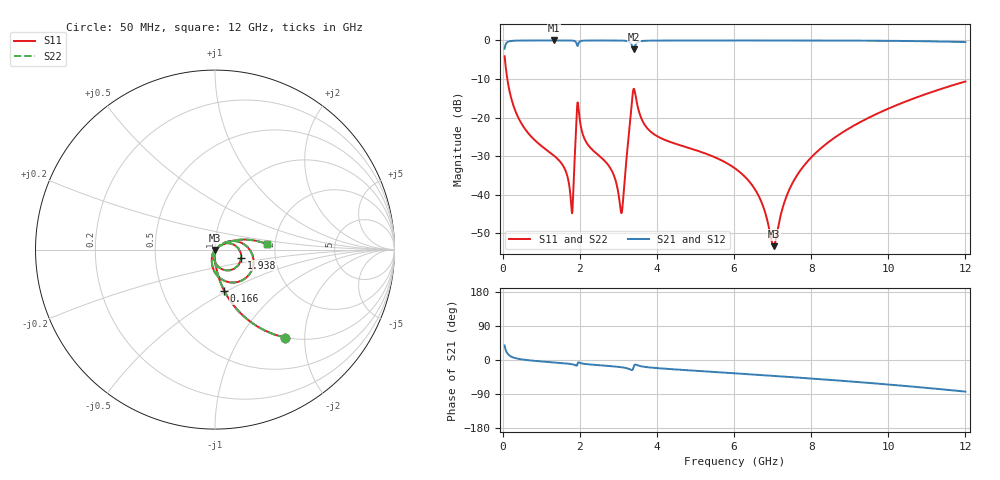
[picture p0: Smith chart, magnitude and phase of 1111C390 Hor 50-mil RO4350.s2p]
# GHz S MA R 50
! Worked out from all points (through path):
!   11951 points, 50 MHz to 12 GHz, reference 50 ohm
!   highest |S21| = -0.01 dB at 1.339 GHz (marker M1); lowest = -2.3 dB at 3.394 GHz (marker M2)
!   group delay of S21, straight-line fit = 19.6 ps
!   lowest |S11| = -53.3 dB at 7.025 GHz (marker M3), VSWR 1.00, Z = 50.2 - j0.147 ohm
!   |S11| at or under -10 dB: 120.3 MHz to end of sweep
!   |S22| runs from -53.3 to -4.1 dB; largest |S21 - S12| = 0
!   S11 on the Smith chart (normalised r, x): 50 MHz: 0.99, -1.59; 166 MHz: 0.99, -0.48; 1.938 GHz: 1.34, -0.12; 12 GHz: 1.82, +0.12
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0.05  0.6251 -51.6  0.7804 38.4  0.7804 38.4  0.6251 -51.6
0.166  0.2351 -77.4  0.9716 12.6  0.9716 12.6  0.2351 -77.4
0.549  0.07494 -88.8  0.9966 0.8  0.9966 0.8  0.07494 -88.8
1.339  0.03189 -95.0  0.9985 -6.6  0.9985 -6.6  0.03189 -95.0
1.624  0.02094 -94.7  0.9981 -9.0  0.9981 -9.0  0.02094 -94.7
1.786  0.006508 -55.1  0.9952 -10.9  0.9952 -10.9  0.006508 -55.1
1.832  0.01139 27.1  0.991 -11.9  0.991 -11.9  0.01139 27.1
1.938  0.1535 -17.1  0.847 -11.2  0.847 -11.2  0.1535 -17.1
2.042  0.07096 -89.1  0.9855 -8.8  0.9855 -8.8  0.07096 -89.1
2.827  0.02066 -99.6  0.9972 -16.4  0.9972 -16.4  0.02066 -99.6
3.074  0.005872 -40.8  0.9944 -19.0  0.9944 -19.0  0.005872 -40.8
3.125  0.008987 15.6  0.9925 -19.7  0.9925 -19.7  0.008987 15.6
3.394  0.2342 -26.9  0.7672 -19.3  0.7672 -19.3  0.2342 -26.9
3.662  0.08397 -101.3  0.9866 -17.9  0.9866 -17.9  0.08397 -101.3
4.034  0.05648 -108.4  0.9949 -21.7  0.9949 -21.7  0.05648 -108.4
6.025  0.02203 -120.0  0.9974 -35.2  0.9974 -35.2  0.02203 -120.0
6.629  0.009901 -117.1  0.9975 -39.2  0.9975 -39.2  0.009901 -117.1
7.025  0.002166 -42.6  0.9975 -41.9  0.9975 -41.9  0.002166 -42.6
7.423  0.0114 33.8  0.9973 -44.7  0.9973 -44.7  0.0114 33.8
8.017  0.03111 36.5  0.9967 -49.0  0.9967 -49.0  0.03111 36.5
10.009  0.1312 23.9  0.9877 -64.7  0.9877 -64.7  0.1312 23.9
12  0.2939 5.8  0.951 -83.4  0.951 -83.4  0.2939 5.8
